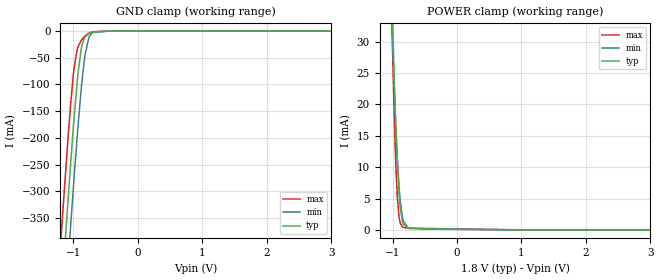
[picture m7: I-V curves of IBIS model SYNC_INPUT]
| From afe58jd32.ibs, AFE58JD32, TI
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|   Model
[Model]   SYNC_INPUT
Model_type   Input
Vinl = 0.45
Vinh = 1.35
|   typ   min   max
C_comp   0.188pF   0.157pF   0.249pF
[Voltage Range]   1.8   1.7   1.9
[Temperature Range]   25   85   -40
[Power Clamp Reference]   1.8   1.7   1.9
[GND Clamp Reference]   -0   -0   -0
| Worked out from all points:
|   GND clamp passes 1 mA (typ) near -0.61 V on its own axis
|   POWER clamp passes 1 mA (typ) near -0.84 V on its own axis
[GND Clamp]
|   Voltage   I(typ)   I(min)   I(max)
-1.8V     -1.671A    -1.791A    -1.551A
-1.195V   -518.2mA   -640.1mA   -395.7mA
-1.174V   -478.8mA   -600.5mA   -356.9mA
-1.087V   -325.2mA   -444.9mA   -207.7mA
-1.039V   -242.7mA   -359.9mA   -132.2mA
-990mV    -165.3mA   -277.7mA   -70.76mA
-941.4mV  -96.78mA   -199.7mA   -34.9mA
-882mV    -36.65mA   -113.9mA   -18.36mA
-817.2mV  -10.9mA    -43.23mA   -9.142mA
-757.8mV  -4.512mA   -11.58mA   -4.051mA
-450mV    -132.6uA   -113.9uA   -164.4uA
3.595V    0A         0A         0A
[POWER Clamp]
|   Voltage   I(typ)   I(min)   I(max)
-1.8V     409.8mA    346.3mA    478.5mA
-1.012V   37.77mA    33.78mA    33.5mA
-1.006V   35.75mA    32.12mA    31.14mA
-973.8mV  24.37mA    22.76mA    18.26mA
-957.6mV  19.27mA    18.55mA    12.89mA
-925.2mV  10.73mA    11.32mA    5.157mA
-898.2mV  5.693mA    6.779mA    1.986mA
-882mV    3.654mA    4.752mA    1.124mA
-844.2mV  1.188mA    1.865mA    444.6uA
-752.4mV  241.2uA    261.7uA    294.9uA
-450mV    172.4uA    131.5uA    237.8uA
3.595V    0A         0A         0A
